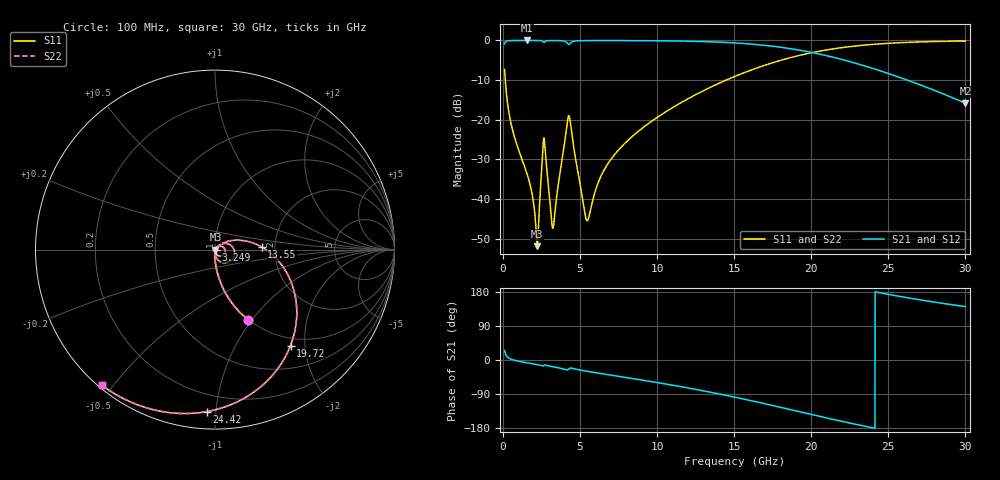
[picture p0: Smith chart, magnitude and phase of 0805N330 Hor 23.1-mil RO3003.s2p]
# GHz S MA R 50
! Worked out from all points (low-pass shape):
!   3201 points, 100 MHz to 30 GHz, reference 50 ohm
!   highest |S21| = -0.01 dB at 1.539 GHz (marker M1); lowest = -15.9 dB at 30 GHz (marker M2)
!   |S21| within 3 dB of the highest: start of sweep to 19.99 GHz
!   lowest |S11| = -51.9 dB at 2.221 GHz (marker M3), VSWR 1.01, Z = 50.2 - j0.0985 ohm
!   |S11| at or under -10 dB: 143 MHz to 14.49 GHz (14.35 GHz wide, 196 % of centre)
!   |S22| runs from -51.9 to -0.1 dB; largest |S21 - S12| = 0
!   S11 on the Smith chart (normalised r, x): 100 MHz: 0.99, -0.95; 3.249 GHz: 1.01, -0.00; 13.55 GHz: 1.70, +0.05; 19.72 GHz: 0.87, -1.72; 24.42 GHz: 0.10, -0.95; 30 GHz: 0.01, -0.47
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0.1  0.4305 -65.0  0.9022 24.9  0.9022 24.9  0.4305 -65.0
0.5671875  0.08089 -88.1  0.9961 1.5  0.9961 1.5  0.08089 -88.1
1.538938  0.02121 -94.3  0.9986 -7.3  0.9986 -7.3  0.02121 -94.3
2.221031  0.002532 -22.8  0.9974 -12.2  0.9974 -12.2  0.002532 -22.8
2.333156  0.006339 40.0  0.9961 -13.2  0.9961 -13.2  0.006339 40.0
2.548062  0.03373 33.3  0.9774 -15.5  0.9774 -15.5  0.03373 33.3
2.660188  0.0585 -23.8  0.9422 -14.1  0.9422 -14.1  0.0585 -23.8
3.118031  0.006246 -58.8  0.9952 -16.9  0.9952 -16.9  0.006246 -58.8
3.248844  0.004319 -6.0  0.9957 -18.0  0.9957 -18.0  0.004319 -6.0
4.248625  0.1119 -13.3  0.8899 -24.6  0.8899 -24.6  0.1119 -13.3
5.089563  0.01202 -80.1  0.9925 -27.3  0.9925 -27.3  0.01202 -80.1
5.500687  0.005398 -11.6  0.9947 -30.2  0.9947 -30.2  0.005398 -11.6
6.164094  0.0159 40.7  0.9956 -34.5  0.9956 -34.5  0.0159 40.7
6.920937  0.03007 43.6  0.9956 -39.3  0.9956 -39.3  0.03007 43.6
10.06978  0.109 27.9  0.9895 -60.0  0.9895 -60.0  0.109 27.9
13.54566  0.261 3.1  0.9594 -85.7  0.9594 -85.7  0.261 3.1
15.05  0.3518 -9.2  0.9294 -98.2  0.9294 -98.2  0.3518 -9.2
19.72188  0.6802 -51.8  0.7239 -141.1  0.7239 -141.1  0.6802 -51.8
20.03956  0.7008 -54.8  0.704 -144.1  0.704 -144.1  0.7008 -54.8
24.42178  0.9037 -92.9  0.4168 177.7  0.4168 177.7  0.9037 -92.9
25.01978  0.9195 -97.5  0.3815 173.1  0.3815 173.1  0.9195 -97.5
30  0.9841 -129.8  0.1611 140.9  0.1611 140.9  0.9841 -129.8
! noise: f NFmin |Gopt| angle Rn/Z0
0.1  0.0004709  0.8716  0.813  0.00079
3.417  0.009237  0.7877  18.81  0.00872
6.743  0.01203  0.7002  36.54  0.007107
10.06  0.0153  0.6651  53.12  0.007076
13.39  0.02005  0.6701  68.59  0.008122
16.7  0.02632  0.6931  82.96  0.009625
20.03  0.03512  0.7294  96.57  0.01179
23.35  0.04836  0.776  109.7  0.0151
26.67  0.07041  0.8299  122.8  0.02058
30  0.112  0.8855  136  0.03051
